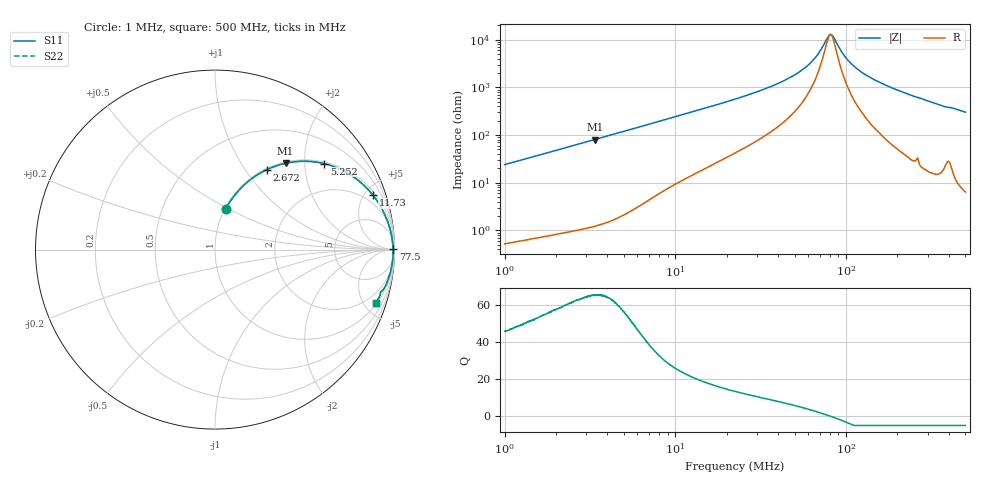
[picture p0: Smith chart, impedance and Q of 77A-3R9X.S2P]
!s-Parameter Generated by FASTRON Sdn. Bhd.
!FASTRON P/N : 77A-3R9X
!Keysight Technologies,E4991B,MY54100416,A.01.15
!Date: Mon May 11 15:33:52 2026
!Version  : Rev00 Mon May 11 15:33:52 2026
!Data & Calibration Information:
!PortZ  Port1:50+j0  Port2:50+j0
!When reading, reference impedance value at option line is always used.
! Remarks : This data is being provided solely for informational purposes.
!Freq	S11	S21	S12	S22
# Hz S dB R 50
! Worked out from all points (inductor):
!   1601 points, 1 MHz to 500 MHz, reference 50 ohm
!   read as one part in series: L = 3.8 uH near 1.032 MHz
!   highest Q = 65.6 at 3.373 MHz (marker M1), where L = 3.79 uH
!   self-resonance near 81.07 MHz
!   S11 on the Smith chart (normalised r, x): 1 MHz: 1.01, +0.48; 2.672 MHz: 1.02, +1.27; 5.252 MHz: 1.05, +2.51; 11.73 MHz: 1.25, +5.68; 77.5 MHz: open; 500 MHz: 1.13, -6.03
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1000000  -12.70 75.4  -0.28 -13.4  -0.28 -13.4  -12.70 75.4
1682824  -8.64 67.3  -0.70 -21.7  -0.70 -21.7  -8.64 67.3
2671620  -5.48 56.9  -1.53 -32.2  -1.53 -32.2  -5.48 56.9
2820919  -5.15 55.5  -1.68 -33.6  -1.68 -33.6  -5.15 55.5
3372764  -4.14 50.7  -2.22 -38.4  -2.22 -38.4  -4.14 50.7
5251551  -2.21 38.1  -4.19 -50.8  -4.19 -50.8  -2.21 38.1
7957584  -1.15 27.2  -6.79 -61.1  -6.79 -61.1  -1.15 27.2
1.173456e7  -0.63 19.1  -9.69 -68.4  -9.69 -68.4  -0.63 19.1
2.236068e7  -0.24 9.9  -15.28 -75.8  -15.28 -75.8  -0.24 9.9
4.344476e7  -0.11 4.1  -22.94 -78.0  -22.94 -78.0  -0.11 4.1
5.358308e7  -0.09 2.6  -26.64 -76.2  -26.64 -76.2  -0.09 2.6
6.307767e7  -0.08 1.6  -30.89 -71.2  -30.89 -71.2  -0.08 1.6
6.950996e7  -0.07 1.0  -34.64 -62.9  -34.64 -62.9  -0.07 1.0
7.749595e7  -0.07 0.3  -40.68 -31.5  -40.68 -31.5  -0.07 0.3
8.02529e7  -0.07 0.1  -42.13 -8.1  -42.13 -8.1  -0.07 0.1
8.310792e7  -0.07 -0.2  -41.83 19.3  -41.83 19.3  -0.07 -0.2
9.821487e7  -0.07 -1.2  -33.04 69.7  -33.04 69.7  -0.07 -1.2
1.16973e8  -0.07 -2.4  -27.62 78.1  -27.62 78.1  -0.07 -2.4
1.409467e8  -0.08 -3.6  -23.88 80.3  -23.88 80.3  -0.08 -3.6
1.77937e8  -0.10 -5.5  -20.41 80.6  -20.41 80.6  -0.10 -5.5
3.443751e8  -0.28 -12.7  -13.16 75.4  -13.16 75.4  -0.28 -12.7
5e8  -0.51 -18.2  -10.09 70.6  -10.09 70.6  -0.51 -18.2
